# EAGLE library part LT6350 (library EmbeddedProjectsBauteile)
LINEAR TECHNOLOGY - LT6350 - OP-VERST, ADC-TREIBER,115MHZ,8MSOP
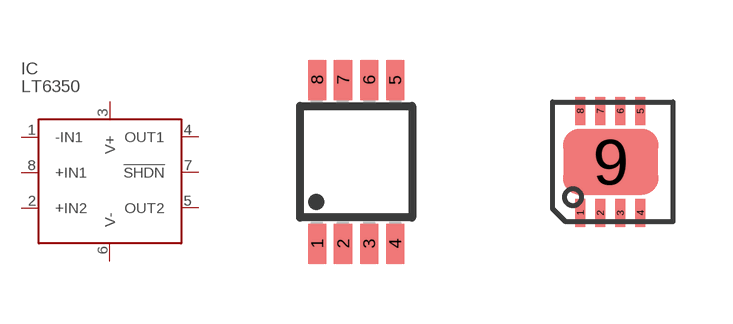
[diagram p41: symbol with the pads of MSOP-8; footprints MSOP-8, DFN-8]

Designator prefix IC

## LT6350CMS8  [MSOP-8]
1  -IN1  in
2  +IN2  in
3  V+  pwr
4  OUT1  pas
5  OUT2  pas
6  V-  pwr
7  !SHDN  in
8  +IN1  in

## LT6350CDD (EP: 401440)  [DFN-8]
1  -IN1  in
2  +IN2  in
3  V+  pwr
4  OUT1  pas
5  OUT2  pas
6  V-  pwr
7  !SHDN  in
8  +IN1  in
9  V-  pwr

## Footprint MSOP-8 (pad centres in mm)
smd 0.45 x 1: 1 -0.975,-2.05; 2 -0.325,-2.05; 3 0.325,-2.05; 4 0.975,-2.05; 5 0.975,2.05; 6 0.325,2.05; 7 -0.325,2.05; 8 -0.975,2.05

## Footprint DFN-8 (pad centres in mm)
smd 0.25 x 0.7: 1 0.688,0.223; 2 1.188,0.223; 3 1.688,0.223; 4 2.188,0.223; 5 2.188,2.777; 6 1.688,2.777; 7 1.188,2.777; 8 0.688,2.777
smd 2.38 x 1.65: 9 1.45,1.5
